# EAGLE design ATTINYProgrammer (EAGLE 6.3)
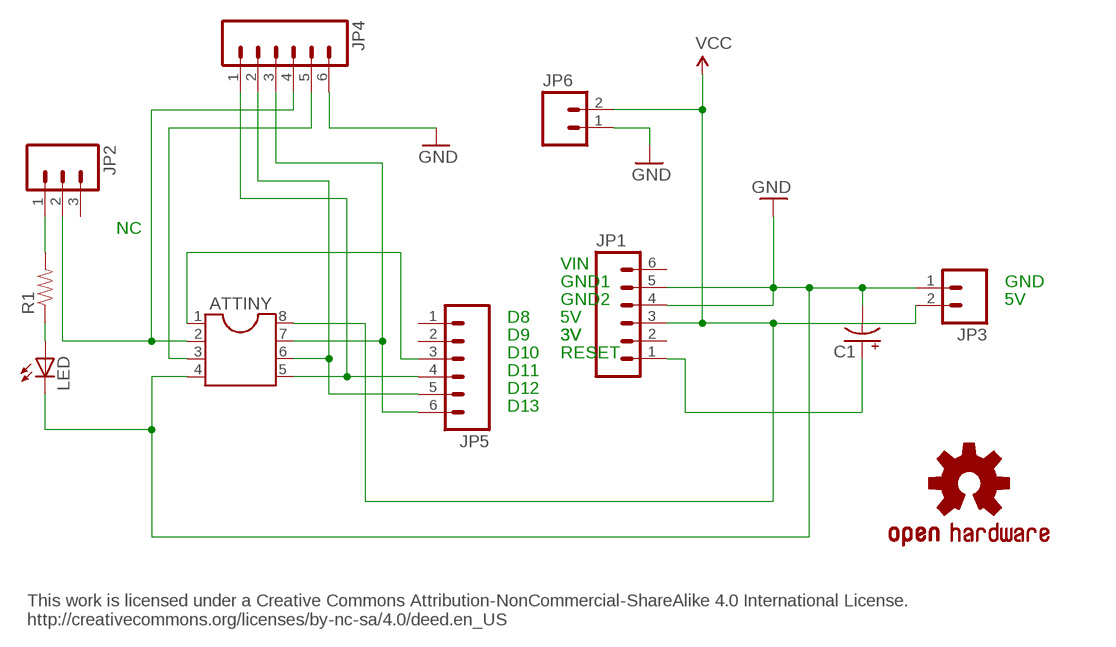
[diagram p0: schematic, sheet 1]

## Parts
ATTINY  DIL8  [DIL08]
C1  CPOL-USE2-5  [E2-5]
JP1  M06SIP  [1X06]
JP2  M03PTH  [1X03]
JP3  M02PTH  [1X02]
JP4  M06SIP  [1X06]
JP5  M06SIP  [1X06]
JP6  M02PTH  [1X02]
LED  LED3MM  [LED3MM]
R1  RESISTORPTH-1/4W  [AXIAL-0.4]
U$2  OSHW-LOGOS  [OSHW-LOGO-S]

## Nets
GND: ATTINY.4 C1.- JP1.4 JP1.5 JP3.1 JP4.6 JP6.1 LED.K(C)
N$1: ATTINY.1 JP5.3
N$2: C1.+ JP1.1
N$4: ATTINY.7 JP4.3 JP5.6
N$5: ATTINY.6 JP4.2 JP5.5
N$6: ATTINY.5 JP4.1 JP5.4
N$7: LED.A R1.P$1
N$8: ATTINY.2 JP2.2 JP4.4
N$9: JP2.1 R1.P$2
N$10: ATTINY.3 JP4.5
VCC: ATTINY.8 JP1.3 JP3.2 JP6.2
Unconnected: JP1.2 JP1.6 JP2.3 JP5.1 JP5.2

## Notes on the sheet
- NC
- VIN
- GND1 | GND
- GND2 | 5V
- D8 | 5V
- D9 | 3V | 3V
- D10 | RESET
- D11
- D12
- D13
- This work is licensed under a Creative Commons Attribution-NonCommercial-ShareAlike 4.0 International License.
  http://creativecommons.org/licenses/by-nc-sa/4.0/deed.en_US

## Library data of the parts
ATTINY = ic-package:DIL8: Dual In Line / Socket
C1 = adafruit:CPOL-US: POLARIZED CAPACITOR, American symbol
JP1 JP4 JP5 = SparkFun:M06: Header 6 Standard 6-pin 0.1" header. Use with straight break away headers (SKU : PRT-00116), right angle break away headers (PRT-00553), swiss pins (PRT-00743), machine pins (PRT-00117), and female headers (PRT-00115). Molex polarized connector foot print use with SKU : PRT-08094 with associated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
JP2 = SparkFun:M03: Header 3 Standard 3-pin 0.1" header. Use with straight break away headers (SKU : PRT-00116), right angle break away headers (PRT-00553), swiss pins (PRT-00743), machine pins (PRT-00117), and female headers (PRT-00115). Molex polarized connector foot print use with SKU : PRT-08232 with associated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
JP3 JP6 = SparkFun:M02: Header 2
LED = adafruit:LED: LED
R1 = SparkFun:RESISTOR: Resistor
U$2 = SparkFun:OSHW-LOGO: Open Source Hardware Logo This logo indicates the piece of hardware it is found on incorporates a OSHW license and/or adheres to the definition of open source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

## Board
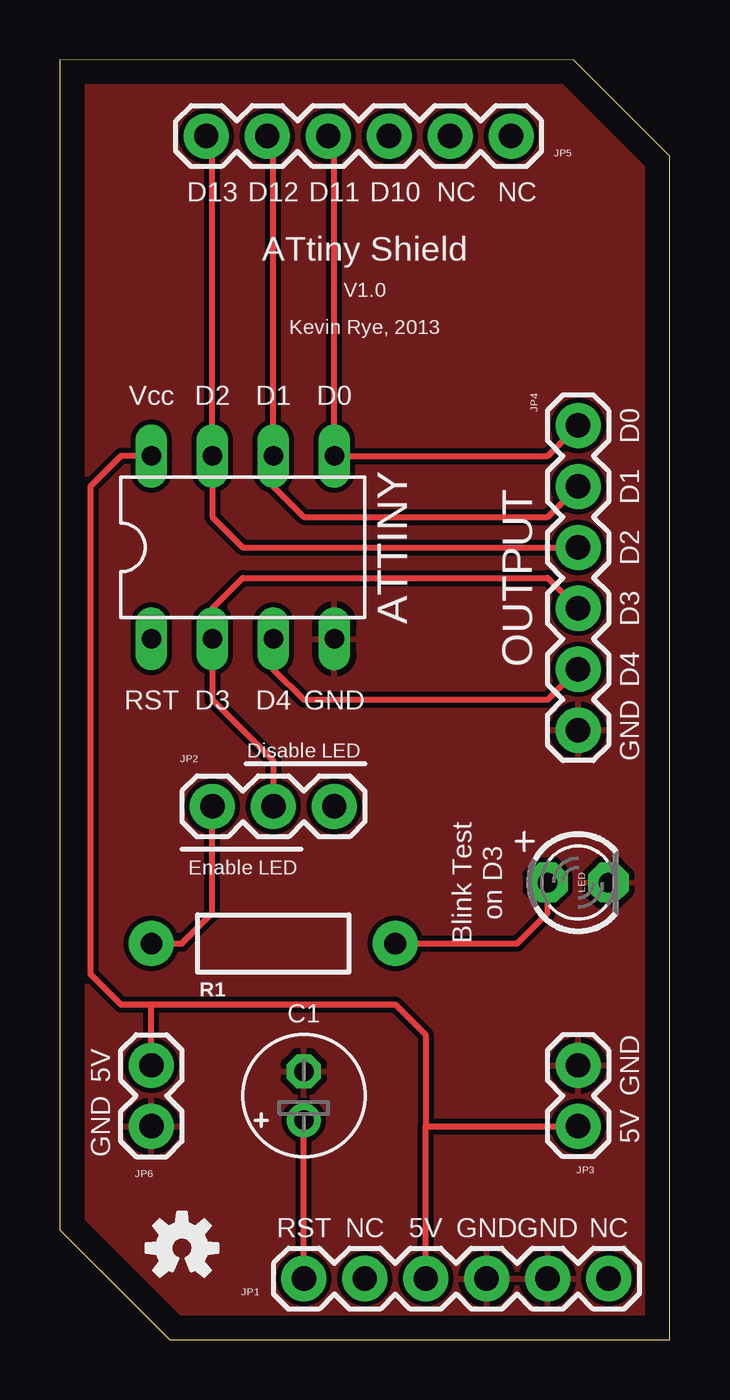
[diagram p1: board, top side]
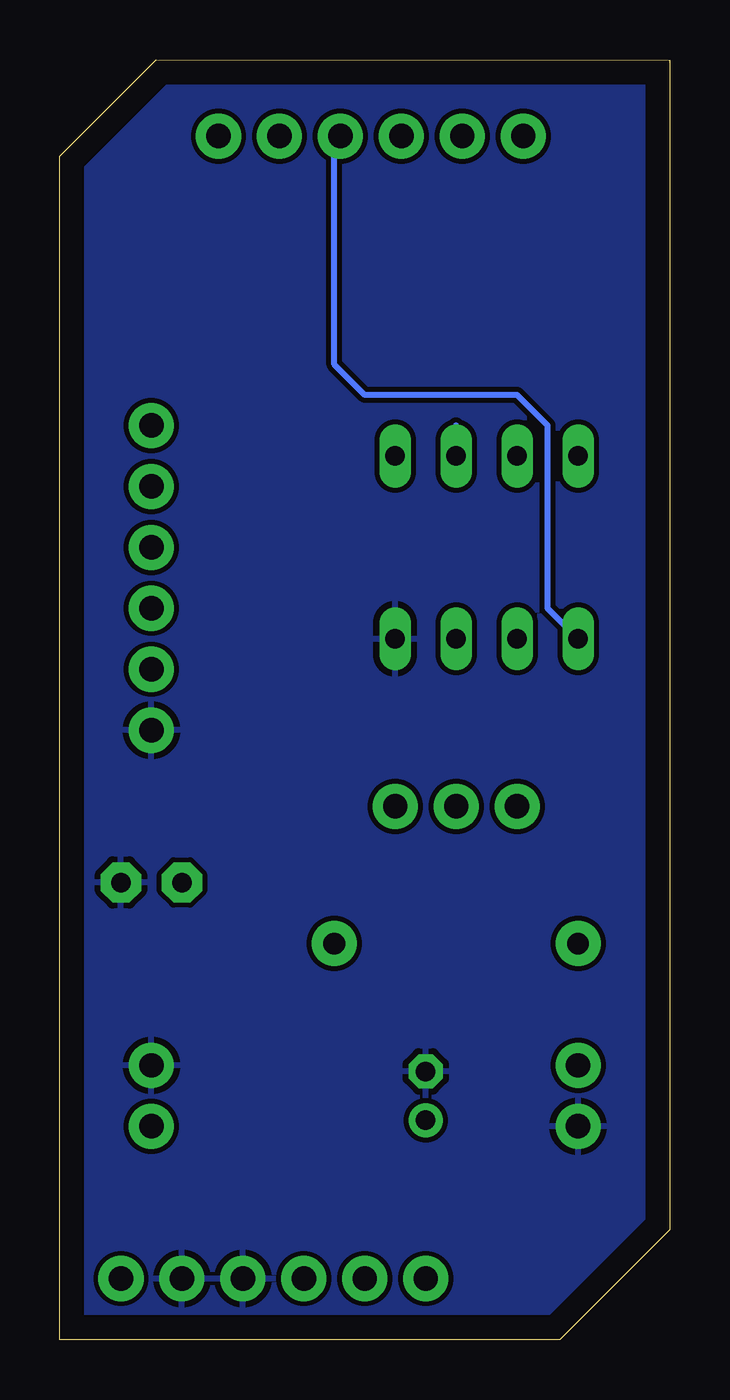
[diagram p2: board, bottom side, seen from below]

Size 25.4 x 53.34 mm. Coordinates in mm from the lower left corner, seen from the top.
Outline: 25.4,49.32 21.38,53.34 0.01,53.33 0,53.32 0,4.58 4.58,0 25.4,0 25.4,49.32
Copper layers (1*16): Top 0.035mm / dielectric 1.5mm / Bottom 0.035mm
Design rules "default": minimum track width 10mil, minimum drill 24mil, track to track 8mil, track to pad 8mil, pad to pad 8mil, via to via 8mil, smd to smd 8mil, copper to edge 40mil, drill to drill 8mil, minimum pad ring 10mil, minimum via ring 8mil, stop-mask expansion 4mil, vias tented up to drill 0mil, thermal gap 10mil

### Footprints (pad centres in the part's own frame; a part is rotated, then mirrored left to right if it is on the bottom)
DIL08 = drill 0.813 long: 1 -3.81,-3.81; 2 -1.27,-3.81; 3 1.27,-3.81; 4 3.81,-3.81; 5 3.81,3.81; 6 1.27,3.81; 7 -1.27,3.81; 8 -3.81,3.81
E2-5 = drill 0.813 pad 1.422: + -1.016,0 | drill 0.813 pad 1.422 octagon: - 1.016,0
1X06 = drill 1.016 pad 1.88: 1 0,0; 2 2.54,0; 3 5.08,0; 4 7.62,0; 5 10.16,0; 6 12.7,0
1X03 = drill 1.016 pad 1.88: 1 0,0; 2 2.54,0; 3 5.08,0
1X02 = drill 1.016 pad 1.88: 1 0,0; 2 2.54,0
LED3MM = drill 0.813 pad 1.676 octagon: A -1.27,0; K 1.27,0
AXIAL-0.4 = drill 0.9 pad 1.88: P$1 -5.08,0; P$2 5.08,0

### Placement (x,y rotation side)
ATTINY  7.62,33.02 0 top
C1  10.16,10.16 90 top
JP1  10.16,2.54 0 top
JP2  6.35,22.23 0 top
JP3  21.59,11.43 270 top
JP4  21.59,38.1 270 top
JP5  18.8,50.16 180 top
JP6  3.81,8.89 90 top
LED  21.59,19.05 0 top
R1  8.89,16.51 180 top
U$2  5.08,3.81 0 top

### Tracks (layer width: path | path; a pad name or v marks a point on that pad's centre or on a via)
GND
  pour Top: -1.27,54.61 26.67,54.61 26.67,-1.27 -1.27,-1.27
  pour Bottom: -1.27,54.61 26.67,54.61 26.67,-1.27 -1.27,-1.27
N$1
  Bottom 0.254: ATTINY.1 5.08,30.48 5.08,38.1 6.35,39.37 12.7,39.37 13.97,40.64 13.97,50.55 JP5.3
N$2
  Top 0.254: JP1.1 C1.+
N$4
  Top 0.254: JP5.6 6.35,50.55 ATTINY.7 6.35,34.29 7.62,33.02 JP4.3
N$5
  Top 0.254: JP5.5 8.89,50.55 ATTINY.6 8.89,35.56 10.16,34.29 20.32,34.29 JP4.2
  Bottom 0.254: ATTINY.6 8.89,38.1
N$6
  Top 0.254: JP5.4 11.43,50.55 ATTINY.5 20.32,36.83 JP4.1
N$7
  Top 0.254: R1.P$1 19.05,16.51 20.32,17.78 LED.A
N$8
  Top 0.254: JP4.4 20.32,31.75 7.62,31.75 6.35,30.48 ATTINY.2 6.35,26.67 8.89,24.13 JP2.2
N$9
  Top 0.254: R1.P$2 5.08,16.51 6.35,17.78 JP2.1
N$10
  Top 0.254: ATTINY.3 8.89,27.94 10.16,26.67 20.32,26.67 JP4.5
VCC
  Top 0.254: ATTINY.8 2.54,36.83 1.27,35.56 1.27,15.24 2.54,13.97 3.81,13.97 | 3.81,13.97 13.97,13.97 15.24,12.7 15.24,8.89 | JP6.2 3.81,13.97 | JP1.3 15.24,8.89 | 15.24,8.89 JP3.2

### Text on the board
Unrouted: This work is licensed under a Creative Commons Attribution-NonCommercial-ShareAlike 4.0 International License. / http://creativecommons.org/licenses/by-nc-sa/4.0/deed.en_US
tNames: D13 | D12 | D11 | D10 | NC | NC | ATtiny Shield | V1.0 | Kevin Rye, 2013 | Vcc | D2 | D1 | D0 | D0 | D1 | D2 | OUTPUT | D3 | D4 | RST | D3 | D4 | GND | GND | Disable LED | Enable LED | Blink Test | on D3 | 5V | GND | GND | 5V | RST | NC | 5V | GND | GND | NC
